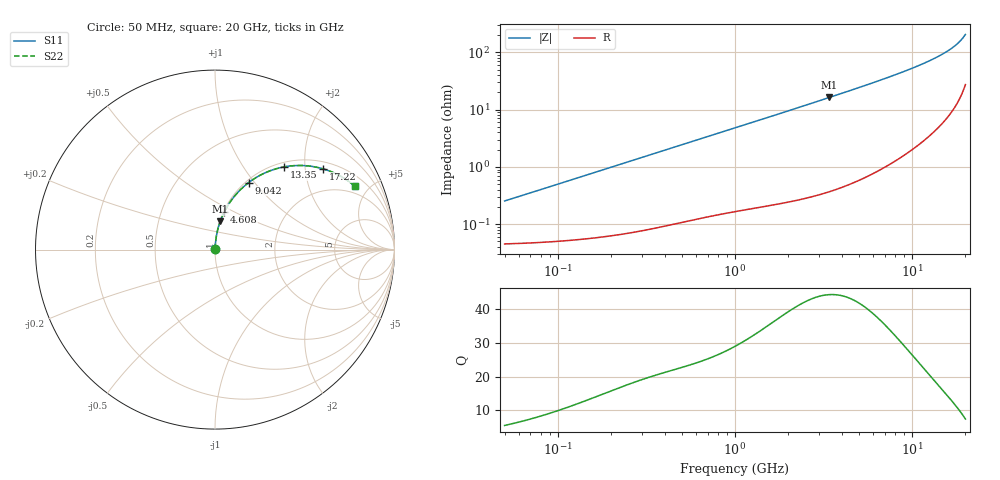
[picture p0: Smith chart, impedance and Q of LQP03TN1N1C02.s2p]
!Murata Part Number: LQP03TN1N1C02
!These Parameters are Measured in Series Mode Connection
!  o--[Z]--o
!Port1  Port2
!  o-------o
!Freq. Start=50[MHz] Stop=20[GHz], 401[Steps]
# Hz S RI R 50
!Freq.(Hz) S11(Real) S11(Imag) S21(Real) S21(Imag) S12(Real) S12(Imag) S22(Real) S22(Imag)
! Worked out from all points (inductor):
!   401 points, 50 MHz to 20 GHz, reference 50 ohm
!   read as one part in series: L = 794 pH near 51.52 MHz
!   highest Q = 44.3 at 3.415 GHz (marker M1), where L = 760 pH
!   S11 on the Smith chart (normalised r, x): 50 MHz: 1.00, +0.00; 4.608 GHz: 1.01, +0.44; 9.042 GHz: 1.03, +0.93; 13.35 GHz: 1.08, +1.56; 17.22 GHz: 1.21, +2.51; 20 GHz: 1.55, +4.07
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5e7  0.000457 0.0025  0.9995 -0.0025  0.9995 -0.0025  0.000457 0.0025
5.388846e7  0.000462 0.00269  0.9995 -0.00269  0.9995 -0.00269  0.000462 0.00269
1.364002e8  0.000589 0.00675  0.9994 -0.00675  0.9994 -0.00675  0.000589 0.00675
3.721004e8  0.00121 0.0181  0.9988 -0.0181  0.9988 -0.0181  0.00121 0.0181
1e9  0.00393 0.0476  0.9961 -0.0476  0.9961 -0.0476  0.00393 0.0476
1.714689e9  0.00878 0.0807  0.9912 -0.0807  0.9912 -0.0807  0.00878 0.0807
2.728004e9  0.0195 0.127  0.9805 -0.127  0.9805 -0.127  0.0195 0.127
3.415248e9  0.0293 0.1578  0.9707 -0.1578  0.9707 -0.1578  0.0293 0.1578
4.608136e9  0.0515 0.2097  0.9485 -0.2097  0.9485 -0.2097  0.0515 0.2097
5.944466e9  0.0838 0.2645  0.9162 -0.2645  0.9162 -0.2645  0.0838 0.2645
7.442007e9  0.1289 0.3207  0.8711 -0.3207  0.8711 -0.3207  0.1289 0.3207
9.041845e9  0.1868 0.3729  0.8132 -0.3729  0.8132 -0.3729  0.1868 0.3729
1.004137e10  0.2278 0.4008  0.7722 -0.4008  0.7722 -0.4008  0.2278 0.4008
1.115139e10  0.2772 0.4269  0.7228 -0.4269  0.7228 -0.4269  0.2772 0.4269
1.220001e10  0.3273 0.4462  0.6727 -0.4462  0.6727 -0.4462  0.3273 0.4462
1.334722e10  0.3856 0.4609  0.6144 -0.4609  0.6144 -0.4609  0.3856 0.4609
1.527346e10  0.4907 0.4683  0.5093 -0.4683  0.5093 -0.4683  0.4907 0.4683
1.621653e10  0.545 0.4628  0.455 -0.4628  0.455 -0.4628  0.545 0.4628
1.721783e10  0.6044 0.4493  0.3956 -0.4493  0.3956 -0.4493  0.6044 0.4493
1.828096e10  0.6695 0.4245  0.3305 -0.4245  0.3305 -0.4245  0.6695 0.4245
1.940974e10  0.7408 0.3831  0.2592 -0.3831  0.2592 -0.3831  0.7408 0.3831
2e10  0.7789 0.3532  0.2211 -0.3532  0.2211 -0.3532  0.7789 0.3532
